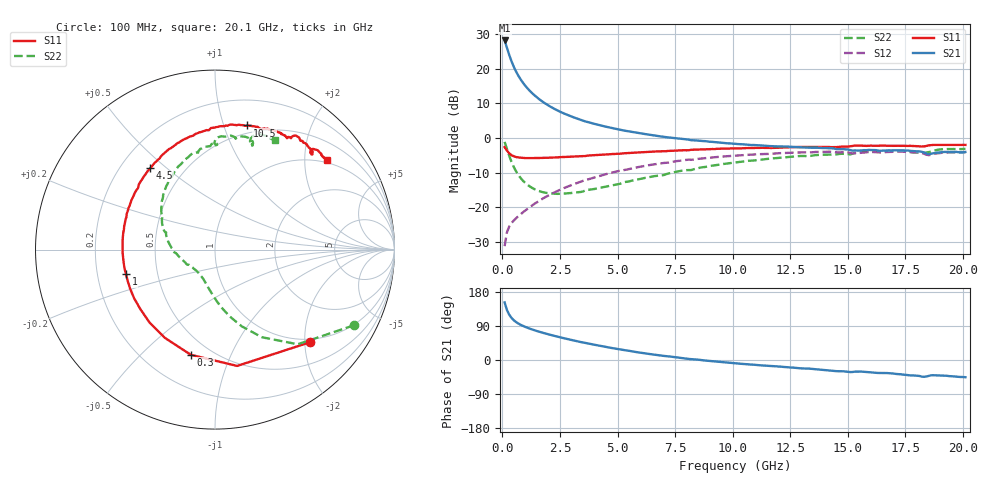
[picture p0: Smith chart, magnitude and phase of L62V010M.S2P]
!  Infineon Technologies AG
! BFR380L3 , PF131585-7, No.6, Th 09.10.01, soldered on pcb-board, measured with PP GSG850
!  Vce=2.0 V,  Ic=10.0 mA
! Common Emitter S-Parameters:  15. November 2001
#  GHz  S  MA  R  50
! f  S11  S21  S12  S22
! GHz  Mag  Ang  Mag  Ang  Mag  Ang  Mag  Ang
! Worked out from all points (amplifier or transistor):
!   201 points, 100 MHz to 20.1 GHz, reference 50 ohm
!   highest |S21| = 28.1 dB at 100 MHz (marker M1)
!   |S21| within 3 dB of that: start of sweep to 244.3 MHz
!   unconditionally stable (mu >= 1): 1.807 GHz to 4.637 GHz
!   at 3.4 GHz: K = 1.03, MAG = 7.9 dB, |S12| = -12.6 dB
!   at 10.1 GHz: K = 0.95, MSG = 1.7 dB, |S12| = -5.1 dB
!   at 20.1 GHz: K = 0.99, MSG = 0.1 dB, |S12| = -4.1 dB
!   S11 on the Smith chart (normalised r, x): 100 MHz: 0.93, -2.10; 300 MHz: 0.39, -0.72; 1 GHz: 0.33, -0.12; 4.5 GHz: 0.32, +0.44; 10.5 GHz: 0.42, +1.20; 20.1 GHz: 0.94, +2.55
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0.1  0.738 -44.5  25.54 152.0  0.02761 68.1  0.8817 -28.6
0.2  0.6598 -79.2  20.11 132.1  0.04359 56.7  0.7006 -48.8
0.3  0.6014 -103.0  15.81 119.6  0.05303 50.8  0.5539 -61.8
0.4  0.5656 -119.5  12.79 111.0  0.05943 48.5  0.4517 -70.9
0.5  0.5457 -132.0  10.62 104.8  0.06481 48.1  0.3808 -77.6
0.6  0.5319 -141.4  9.061 100.1  0.06996 48.6  0.3305 -82.9
0.7  0.5261 -148.7  7.89 96.1  0.07483 49.4  0.2927 -87.4
0.8  0.5209 -154.8  6.976 92.8  0.0801 50.4  0.2642 -91.2
1  0.5142 -164.4  5.664 87.3  0.09038 52.3  0.2245 -97.9
1.2  0.514 -172.0  4.769 82.5  0.1014 53.9  0.1997 -103.8
1.4  0.515 -178.1  4.123 78.4  0.1129 55.0  0.1829 -109.1
1.6  0.5157 176.5  3.633 74.6  0.1247 55.8  0.1721 -114.0
1.9  0.5198 169.5  3.097 69.4  0.1425 56.3  0.1621 -120.8
2.6  0.5316 156.1  2.321 58.5  0.185 55.7  0.1578 -135.2
3.5  0.5489 141.7  1.783 46.2  0.2413 52.5  0.1693 -150.0
4.5  0.5794 128.5  1.456 34.4  0.3018 47.6  0.1993 -166.9
6.8  0.6427 103.4  1.064 12.4  0.4287 33.1  0.2879 161.7
10.1  0.7093 77.9  0.827 -8.7  0.557 11.7  0.4447 127.8
10.5  0.7149 75.4  0.81 -10.5  0.5691 9.0  0.4615 124.0
13.5  0.7415 60.1  0.7251 -23.8  0.6251 -9.4  0.5606 99.1
16.8  0.7748 48.0  0.6654 -35.0  0.63 -25.4  0.6455 77.5
20.1  0.7962 38.7  0.6297 -45.4  0.6222 -39.1  0.6974 61.1
